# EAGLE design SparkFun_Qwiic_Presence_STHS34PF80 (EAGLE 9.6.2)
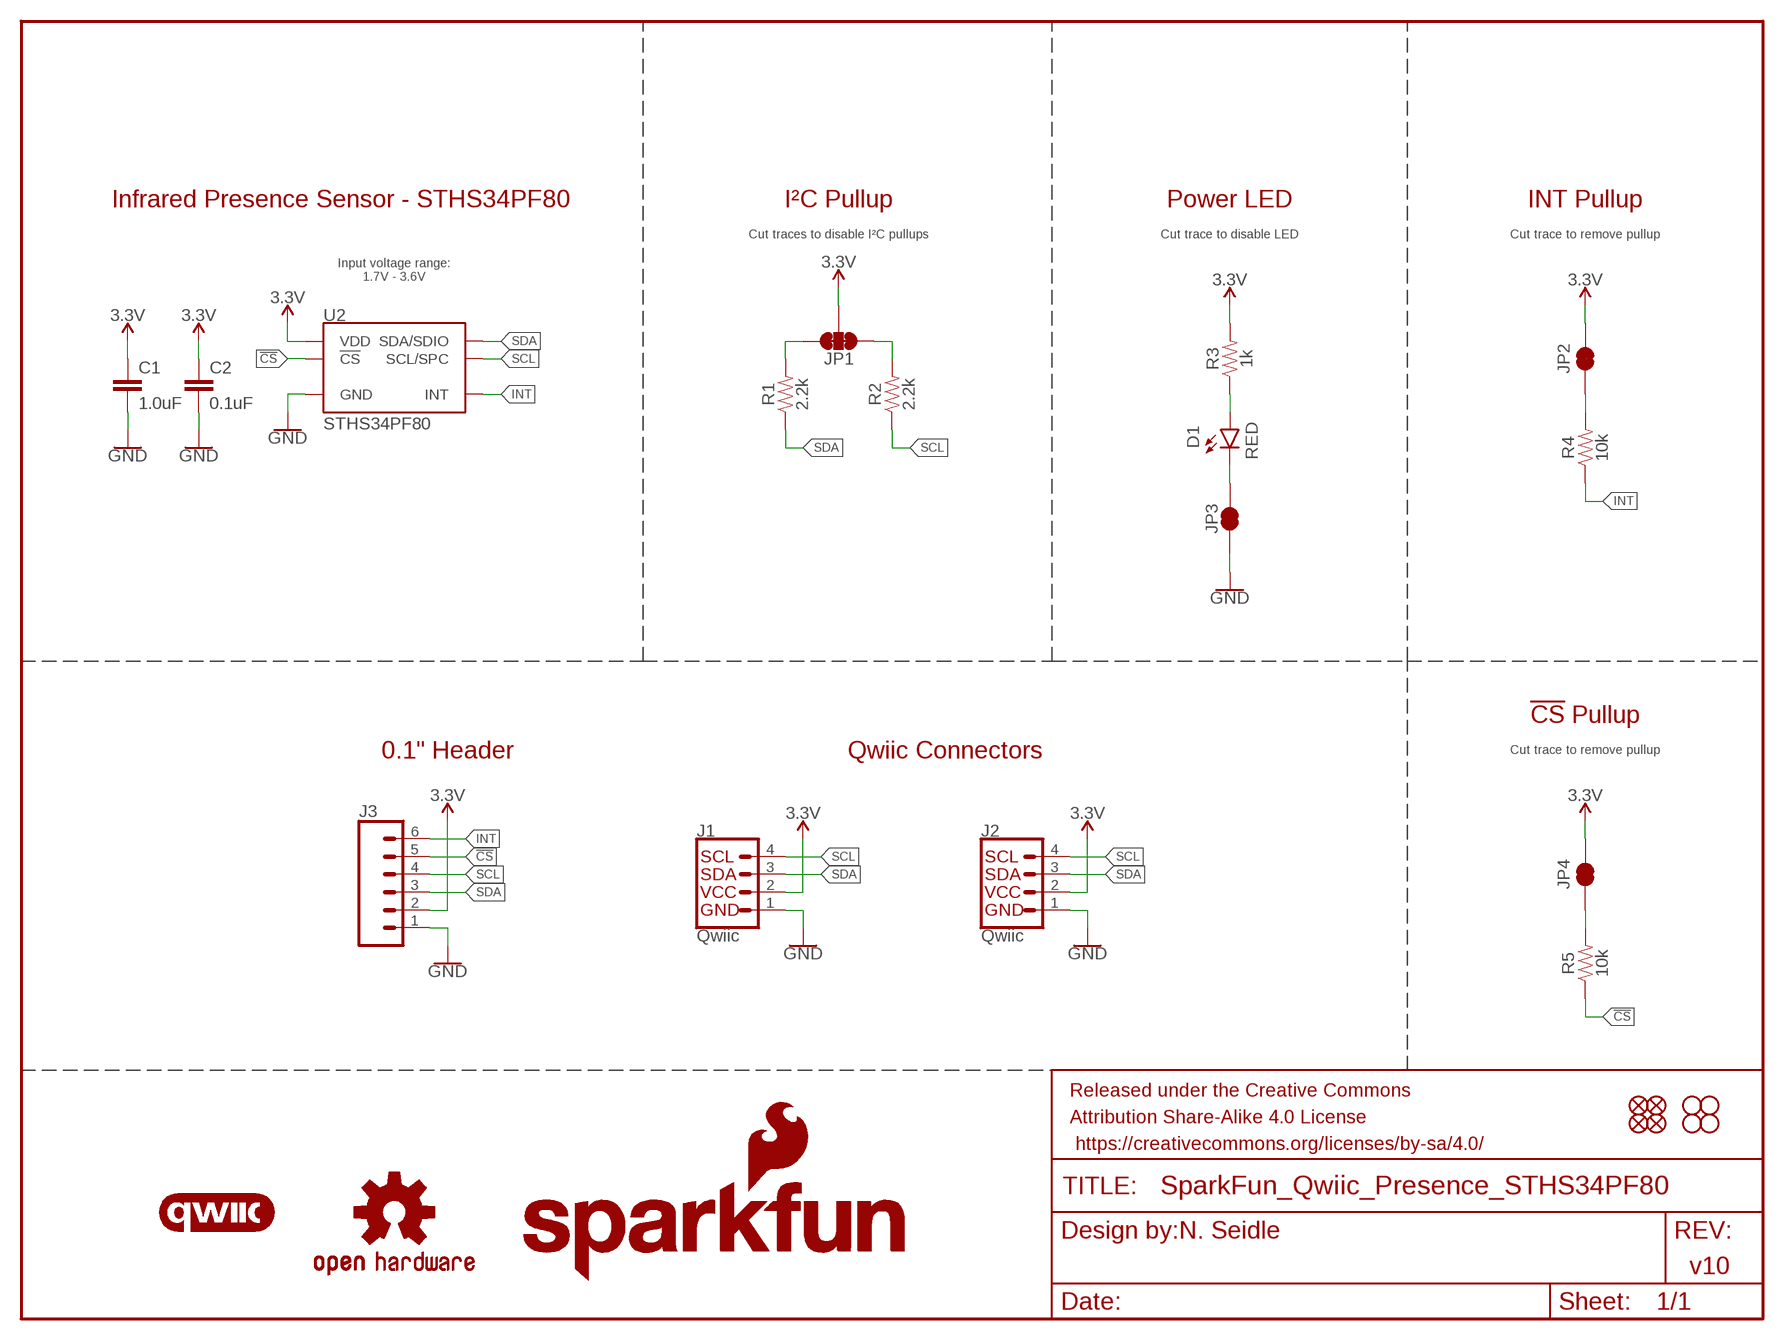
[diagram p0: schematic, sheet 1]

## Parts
C1  1.0uF  1.0UF-0603-16V-10%  [0603]
C2  0.1uF  0.1UF-0603-25V-(+80/-20%)  [0603]
D1  RED  LED-RED0603  [LED-0603]
FD1  FIDUCIAL1X2  [FIDUCIAL-1X2]
FD2  FIDUCIAL1X2  [FIDUCIAL-1X2]
FD3  FIDUCIAL1X2  [FIDUCIAL-1X2]
FD4  FIDUCIAL1X2  [FIDUCIAL-1X2]
FRAME2  FRAME-LETTER  [CREATIVE_COMMONS]
H1  STAND-OFF  [STAND-OFF]
H2  STAND-OFF  [STAND-OFF]
H3  STAND-OFF  [STAND-OFF]
H4  STAND-OFF  [STAND-OFF]
J1  Qwiic  QWIIC_CONNECTORJS-1MM  [JST04_1MM_RA]
J2  Qwiic  QWIIC_CONNECTORJS-1MM  [JST04_1MM_RA]
J3  CONN_06NO_SILK_NO_POP  [1X06_NO_SILK]
JP1  JUMPER-SMT_3_2-NC_TRACE_SILK  [SMT-JUMPER_3_2-NC_TRACE_SILK]
JP2  JUMPER-SMT_2_NC_TRACE_SILK  [SMT-JUMPER_2_NC_TRACE_SILK]
JP3  JUMPER-SMT_2_NC_TRACE_SILK  [SMT-JUMPER_2_NC_TRACE_SILK]
JP4  JUMPER-SMT_2_NC_TRACE_SILK  [SMT-JUMPER_2_NC_TRACE_SILK]
LOGO1  OSHW-LOGOS  [OSHW-LOGO-S]
LOGO2  SFE_LOGO_NAME_FLAME.1_INCH  [SFE_LOGO_NAME_FLAME_.1]
LOGO3  QWIIC_LOGO_CONNECTOR  [QWIIC_5.5MM]
LOGO4  SFE_LOGO_NAME8_MM  [SFE_LOGO_NAME_8MM]
LOGO6  SFE_LOGO_FLAME.1_INCH  [SFE_LOGO_FLAME_.1]
R1  2.2k  2.2KOHM-0603-1/10W-1%  [0603]
R2  2.2k  2.2KOHM-0603-1/10W-1%  [0603]
R3  1k  1KOHM-0603-1/10W-1%  [0603]
R4  10k  10KOHM-0603-1/10W-1%  [0603]
R5  10k  10KOHM-0603-1/10W-1%  [0603]
U2  STHS34PF80  [OLGA-10L]

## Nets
3.3V: C1.1 C2.1 J1.2 J2.2 J3.2 JP1.2 JP2.2 JP4.2 R3.2 U2.6(VDD) U2.9(VDD)
!CS!: J3.5 R5.1 U2.3(!CS!)
GND: C1.2 C2.2 J1.1 J2.1 J3.1 JP3.1 U2.2(GND) U2.7(GND) U2.8(GND)
INT: J3.6 R4.1 U2.10(INT)
N$1: D1.C JP3.2
N$2: JP1.3 R1.2
N$3: JP1.1 R2.2
N$4: D1.A R3.1
N$5: JP2.1 R4.2
N$6: JP4.1 R5.2
SCL: J1.4 J2.4 J3.4 R2.1 U2.1(SCL/SPC)
SDA: J1.3 J2.3 J3.3 R1.1 U2.4(SDA/SDIO)

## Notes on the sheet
- Infrared Presence Sensor - STHS34PF80 | I²C Pullup | Power LED | INT Pullup
- Cut traces to disable I²C pullups | Cut trace to disable LED | Cut trace to remove pullup
- Input voltage range:
  1.7V - 3.6V
- !CS! Pullup
- 0.1" Header | Qwiic Connectors | Cut trace to remove pullup
- N. Seidle
- v10

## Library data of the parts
C1 = SparkFun-Capacitors:1.0UF: 1µF ceramic capacitors; PROD_ID: CAP-00868
C2 = SparkFun-Capacitors:0.1UF: 0.1µF ceramic capacitors; PROD_ID: CAP-00810
D1 = SparkFun-LED:LED-RED: Red SMD LED; PROD_ID: DIO-00819
FD1-FD4 = SparkFun-Aesthetics:FIDUCIAL: Fiducial Alignment Points
FRAME2 = SparkFun-Aesthetics:FRAME-LETTER: Schematic Frame - Letter
H1-H4 = SparkFun-Hardware:STAND-OFF: Stand Off
J1 J2 = SparkFun-Connectors:QWIIC_CONNECTOR: SparkFun I2C Standard Qwiic Connector An SMD 1mm pitch JST connector makes it easy and quick (get it? Qwiic?) to connect I2C devices to each other. The Qwiic system enables fast and solderless connection between popular platforms and various sensors and actuators. We carry 200mm, 100mm, 50mm, and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; PROD_ID: CONN-13694; VALUE: QWIIC_RIGHT_ANGLE
J3 = SparkFun-Connectors:CONN_06: Multi connection point. Often used as Generic Header-pin footprint for 0.1 inch spaced/style header connections On any of the 0.1 inch spaced packages, you can populate with these: Break Away Headers - Straight (PRT-00116) Break Away Male Headers - Right Angle (PRT-00553) Female Headers (PRT-00115)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
JP1 = SparkFun-Jumpers:JUMPER-SMT_3_2-NC_TRACE: Normally closed trace jumper (2 of 2 connections) This jumper has a trace between all three pads so they are normally closed (NC). Use a razor knife to open the connection(s). For best results follow the IPC guidelines for cutting traces: Cutout at least 0.063 mm (0.005 in). Remove all loose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
JP2-JP4 = SparkFun-Jumpers:JUMPER-SMT_2_NC_TRACE: Normally closed trace jumper
LOGO1 = SparkFun-Aesthetics:OSHW-LOGO: Open-Source Hardware (OSHW) Logo
LOGO2 = SparkFun-Aesthetics:SFE_LOGO_NAME_FLAME: SparkFun Font Logo w/ Flame
LOGO3 = SparkFun-Aesthetics:QWIIC_LOGO: Qwiic Logos for placement on schematic and PCB. The 5.5mm silk logo is best for placing next to Qwiic connector.
LOGO4 = SparkFun-Aesthetics:SFE_LOGO_NAME: SparkFun Font Logo
LOGO6 = SparkFun-Aesthetics:SFE_LOGO_FLAME: SparkFun Flame Logo
R1 R2 = SparkFun-Resistors:2.2KOHM: 2.2kΩ resistor; PROD_ID: RES-08272
R3 = SparkFun-Resistors:1KOHM: 1kΩ resistor; PROD_ID: RES-07856
R4 R5 = SparkFun-Resistors:10KOHM: 10kΩ resistor; PROD_ID: RES-00824
U2 = STHS34PF80:STHS34PF80: Bosch BMP384 Pressure Sensor Senses pressure from 300 hPa to 1250 hPa, sends data out over I2C or SPI; PROD_ID: IC-

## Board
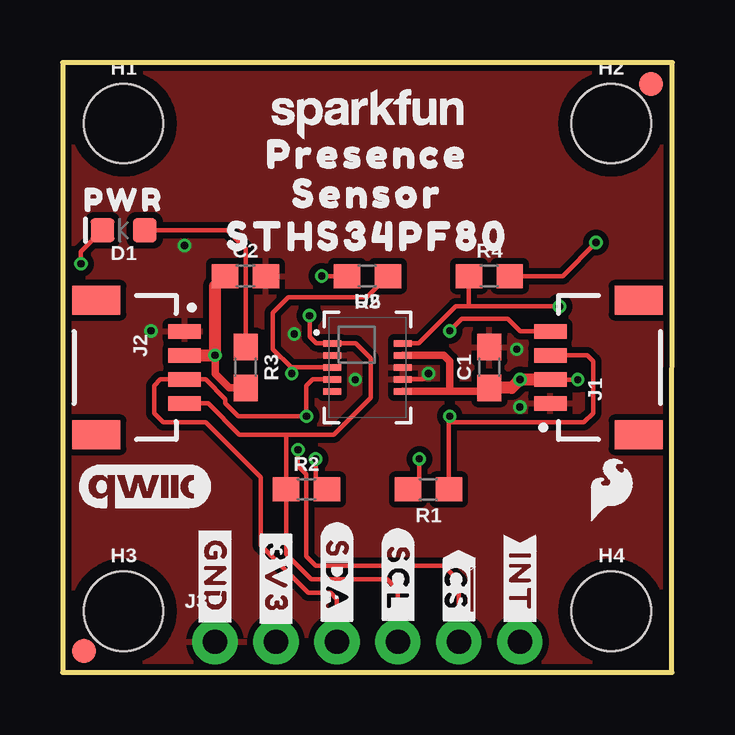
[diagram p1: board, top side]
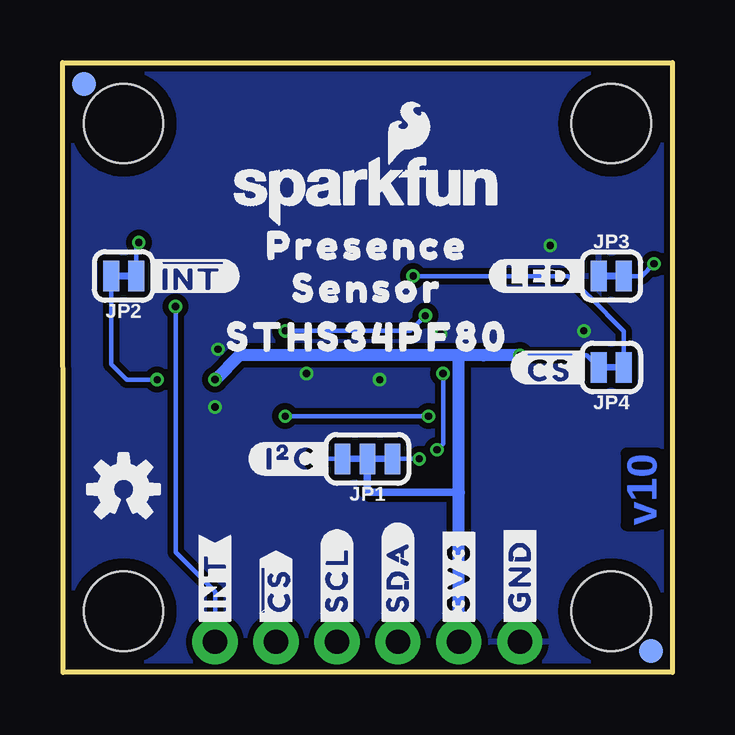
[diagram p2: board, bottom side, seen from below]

Size 25.4 x 25.4 mm. Coordinates in mm from the lower left corner, seen from the top.
Outline: 0,0 25.38,0 25.4,25.4 0,25.4 0,0
Copper layers (1*16): Top 0.035mm / dielectric 1.5mm / Bottom 0.035mm
Design rules "SparkFun-2-Layer-Minimum-JLCPCB": minimum track width 5mil, minimum drill 0.3mm, track to track 5mil, track to pad 5mil, pad to pad 5mil, via to via 5mil, smd to smd 5mil, copper to edge 7mil, drill to drill 7mil, minimum pad ring 5mil, minimum via ring 5mil, stop-mask expansion 2.5mil, vias tented up to drill 25mil, thermal gap 10mil

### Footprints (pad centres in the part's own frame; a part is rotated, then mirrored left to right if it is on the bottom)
0603 = smd 1.1 x 1: 1 -0.85,0; 2 0.85,0
LED-0603 = smd 1 x 1: A -0.877,0; C 0.877,0
FIDUCIAL-1X2 = smd 1 x 1: 1 0,0
STAND-OFF = hole 3.302: 0,0
JST04_1MM_RA = smd 0.6 x 1.35: 1 -1.5,0; 2 -0.5,0; 3 0.5,0; 4 1.5,0 | smd 1.2 x 2: NC1 2.8,-3.675; NC2 -2.8,-3.675
1X06_NO_SILK = drill 1.016 pad 1.88: 1 0,0; 2 2.54,0; 3 5.08,0; 4 7.62,0; 5 10.16,0; 6 12.7,0
SMT-JUMPER_3_2-NC_TRACE_SILK = smd 0.66 x 1.27: 1 -1.041,0; 2 0,0; 3 1.041,0
SMT-JUMPER_2_NC_TRACE_SILK = smd 0.66 x 1.27: 1 -0.521,0; 2 0.521,0
OLGA-10L = smd 0.75 x 0.285: 1 -1.475,1; 2 -1.475,0.5; 3 -1.475,0; 4 -1.475,-0.5; 5 -1.475,-1; 6 1.475,-1; 7 1.475,-0.5; 8 1.475,0; 9 1.475,0.5; 10 1.475,1

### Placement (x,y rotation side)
C1  17.78,12.7 90 top
C2  7.62,16.51 0 top
D1  2.54,18.41 180 top
FD1  0.89,0.89 0 bottom
FD2  0.89,0.89 0 top
FD3  24.51,24.51 0 bottom
FD4  24.51,24.51 0 top
FRAME2  not placed on the board
H1  2.54,22.86 0 top
H2  22.86,22.86 0 top
H3  2.54,2.54 0 top
H4  22.86,2.54 0 top
J1  20.32,12.7 90 top
J2  5.08,12.7 270 top
J3  6.35,1.27 0 top
JP1  12.7,8.89 180 bottom
JP2  22.86,16.51 180 bottom
JP3  2.54,16.51 0 bottom
JP4  2.54,12.7 180 bottom
LOGO1  22.86,7.62 0 bottom
LOGO2  12.7,20.07 0 bottom
LOGO3  3.43,7.75 0 top
LOGO4  12.7,23.37 0 top
LOGO6  22.86,7.62 0 top
R1  15.24,7.62 180 top
R2  10.16,7.62 0 top
R3  7.62,12.7 270 top
R4  17.78,16.51 0 top
R5  12.7,16.51 180 top
U2  12.7,12.7 0 top
U$1  [#I�C#0]  17.65,8.89 0 bottom
U$2  [##CS##0]  16.51,1.78 90 bottom
U$3  [#3V3#0]  8.89,1.78 90 bottom
U$4  [#INT#1]  19.05,1.78 90 bottom
U$5  [STHS34PF800]  12.7,18.16 0 top
U$6  [STHS34PF800]  12.7,13.97 0 bottom
U$7  [PRESENCE0]  12.7,21.59 0 top
U$8  [PRESENCE0]  12.7,17.78 0 bottom
U$9  [PWR11]  2.54,19.68 0 top
U$10  [##INT##0]  21.97,16.51 0 bottom
U$11  [#SDA#0]  11.43,6.22 270 top
U$12  [SENSOR1]  12.7,19.94 0 top
U$13  [##CS##1]  16.51,5.08 270 top
U$14  [SENSOR1]  12.7,16 0 bottom
U$15  [#INT#2]  19.05,5.71 270 top
U$16  [#GND#4]  6.35,6.22 270 top
U$17  [#LED#10]  3.43,16.51 0 bottom
U$18  [#GND#4]  6.35,1.78 90 bottom
U$19  [#3V3#0]  8.89,6.1 270 top
U$20  [#SDA#5]  11.43,1.78 90 bottom
U$21  [#SCL#6]  13.97,1.78 90 bottom
U$22  [#SCL#0]  13.97,5.97 270 top
U$23  [##CS#0]  6.73,12.7 0 bottom

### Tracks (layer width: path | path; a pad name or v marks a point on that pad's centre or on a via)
3.3V  (via drill 0.3)
  Top 0.178: v21.46,12.19 J1.2
  Top 0.305: U2.6 16.13,11.7 | 16.13,11.7 17.63,11.7 C1.1 | U2.9 15.88,13.2 16.13,12.95 16.13,11.7 | R3.2 6.95,11.85 6.35,12.45 v6.35,13.21
  Top 0.508: J2.2 v6.35,13.21 6.35,16.09 C2.1 | J1.2 v19.06,12.2 v19.05,12.19 18.71,11.85 C1.1
  Bottom 0.178: JP2.2 23.38,12.84 22.73,12.19 v21.46,12.19 | JP4.2 3.57,13.21 v6.35,13.21
  Bottom 0.305: JP1.2 12.7,7.62 12.57,7.49 8.89,7.49
  Bottom 0.508: v6.35,13.21 7.87,13.21 8.76,13.21 | 8.76,13.21 18.03,13.21 v19.05,12.19 | J3.2 8.89,7.49 8.89,13.08 8.76,13.21
!CS!  (via drill 0.3)
  Top 0.178: U2.3 9.65,12.7 | v9.8,9.27 9.8,8.61 10.16,8.26 10.16,4.83 10.54,4.45 15.88,4.45 16.51,3.81 J3.5 | 9.65,12.7 9.53,12.7 8.76,13.46 8.76,14.99 9.4,15.62 12.66,15.62 R5.1 | v9.55,12.45 9.55,12.6 9.65,12.7
  Bottom 0.178: v9.55,12.45 9.55,9.53 v9.8,9.27
GND  (via drill 0.3)
  Top 0.178: U2.7 14.99,12.2 v15.24,12.45
  other vias: 3.68,14.22 9.65,14.1 18.92,13.46 19.05,11.05 5.08,17.78 12.19,12.19
  pour Top (isolate 0.254): 0,0 0,25.4 25.4,25.4 25.4,0
  pour Bottom (isolate 0.254): 0,25.4 25.4,25.4 25.4,0 0,0
INT  (via drill 0.3)
  Top 0.178: U2.10 14.84,13.7 16.38,15.24 16.89,15.24 | v20.7,15.24 16.89,15.24 | 16.89,15.24 16.93,15.28 R4.1
  Bottom 0.178: J3.6 19.05,3.36 20.69,5 20.69,15.23 v20.7,15.24
N$1  (via drill 0.3)
  Top 0.178: v0.76,17.02 0.76,17.51 D1.C
  Bottom 0.178: JP3.2 1.27,16.51 v0.76,17.02
N$2  (via drill 0.3)
  Top 0.178: v14.86,8.89 14.86,8.09 R1.2
  Bottom 0.178: JP1.3 v14.86,8.89
N$3  (via drill 0.3)
  Top 0.178: v10.54,8.89 10.54,8.09 R2.2
  Bottom 0.178: JP1.1 v10.54,8.89
N$4
  Top 0.178: D1.A 5.46,18.41 6.86,18.41 7.62,17.65 R3.1
N$5  (via drill 0.3)
  Top 0.178: R4.2 20.83,16.51 v22.23,17.91
  Bottom 0.178: JP2.1 22.34,17.79 v22.23,17.91
N$6  (via drill 0.3)
  Top 0.178: R5.2 v10.79,16.51
  Bottom 0.178: v10.79,16.51 4.33,16.51 3.48,15.66 3.47,15.66 2.02,14.21 JP4.1
SCL  (via drill 0.3)
  Top 0.178: J2.4 6.07,11.2 7.37,9.91 9.27,9.91 | 9.27,9.91 11.3,9.91 12.83,11.43 12.83,13.08 12.21,13.7 U2.1 10.56,13.7 10.29,13.97 v10.29,14.86 | J1.4 19.07,14.2 18.54,14.73 16.64,14.73 v16.13,14.22 | J3.4 13.97,3.43 13.53,3.87 10.35,3.87 9.31,4.91 R2.1 9.31,9.87 9.27,9.91
  Bottom 0.178: v16.13,14.22 10.92,14.22 v10.29,14.86
SDA  (via drill 0.3)
  Top 0.178: J1.3 21.85,13.2 22.1,12.95 22.1,10.79 21.72,10.41 16.22,10.41 16.09,10.54 | R1.1 16.09,10.54 | 16.09,10.54 16.09,10.63 v16.13,10.67 | U2.4 10.42,12.2 10.16,11.94 v10.16,10.67 7.32,10.67 6.78,11.21 6.78,11.38 5.96,12.2 J2.3 4.07,12.2 3.81,11.94 3.81,10.79 4.19,10.41 5.97,10.41 8.26,8.13 8.26,5.28 10.22,3.31 11.16,3.31 11.43,3.05 J3.3
  Bottom 0.178: v16.13,10.67 v10.16,10.67

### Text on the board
Bottom: v10
Measures: Units: inches
tDocu: N. Seidle

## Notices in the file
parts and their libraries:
SparkFun-PowerSymbols: Licensing: Creative Commons ShareAlike 4.0 International - https://creativecommons.org/licenses/by-sa/4.0
SparkFun-Aesthetics: Released under the Creative Commons Attribution Share-Alike 4.0 License
SparkFun-Aesthetics: https://creativecommons.org/licenses/by-sa/4.0
